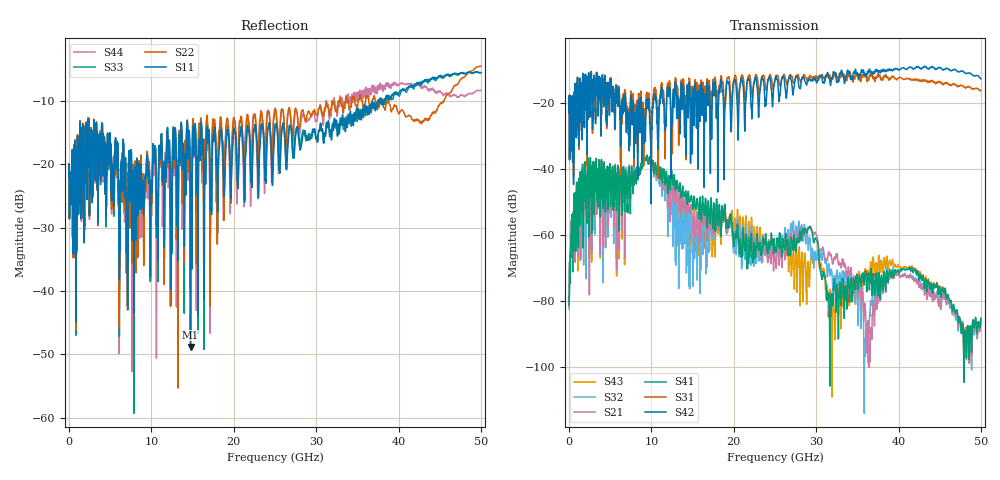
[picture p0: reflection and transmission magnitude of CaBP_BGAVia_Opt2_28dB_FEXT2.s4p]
!* Samtec Inc. NovaRay Examax Flyover System  *
!*  REV DATE  = 08/08/18  *
!*  TYPE  = TOUCHSTONE  *
!*  PORTS  = 4 port  *
!*  UNITS  = GHz  *
!*  DATA RANGE = DC  to 50 GHz; 10 MHz Step  *
!*  PARAMETER  = S  *
!*  FORMAT  = Real-Imaginary  *
!*  REFERENCE  = 50 ohms  *
!*  SOURCE  = HFSS  *
!*  VALIDATED  = No  *
!*  MANUFACTURER = SAMTEC  *
!*  INTERCONNECT = NVAx to EBCx to EBCx to NVAx  *
!*  [Full Channel NVAx to EBCx to EBCx to NVAx  with PCB Trace and BGA Via]  *
!*  BOUNDARY A  = Silicon BGA Ball Pad  *
!*  BOUNDARY B  = Silicon BGA Ball Pad  *
!*  NVAx (end a) ->>- (end b) NVAx  *
!*  Port 01 ->>- Port 02  *
!*  Port 03 ->>- Port 04  *
!***************************** CHANNEL MODEL ******************************************
# GHz S RI R 50
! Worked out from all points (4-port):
!   5000 points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, 10 MHz to 50 GHz, reference 50 ohm
!   strongest paths, dB at 10 MHz, 12.51 GHz, 25.01 GHz, 37.51 GHz, 50 GHz:
!     S42: -23.1, -26.3, -12.7, -10.5, -12.7
!     S31: -23.1, -28.5, -13.0, -11.3, -16.4
!     S41: -81.3, -42.6, -64.0, -77.3, -85.4
!     S21: -82.1, -46.0, -67.1, -78.8, -86.3
!     S32: -82.7, -51.9, -65.2, -75.4, -86.3
!     S43: -81.6, -46.4, -64.4, -70.1, -85.3
!   lowest |S11| = -48.8 dB at 14.75 GHz (marker M1), VSWR 1.01, Z = 49.7 - j0.221 ohm
!   |S11| at or under -10 dB: start of sweep to 37.51 GHz; 37.83997 GHz to 38.00552 GHz (165.6 MHz wide, 0.437 % of centre); 38.04261 GHz to 38.22467 GHz (182.1 MHz wide, 0.477 % of centre)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
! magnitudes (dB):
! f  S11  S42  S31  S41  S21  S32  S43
! 10 MHz  -22.1  -23.1  -23.1  -81.3  -82.1  -82.7  -81.6
! 1.43 GHz  -14.9  -13.9  -13.8  -48.1  -50.2  -52.2  -50.2
! 9.26 GHz  -21.6  -31.8  -26.8  -37.1  -37.3  -37.3  -37.0
! 14.75 GHz  -48.8  -38.3  -22.0  -49.3  -51.7  -56.3  -55.7
! 29.25 GHz  -16.1  -12.7  -11.7  -57.6  -57.7  -61.1  -71.4
! 31.79 GHz  -15.2  -14.1  -13.4  -78.6  -66.1  -71.1  -78.7
! 50 GHz  -5.6  -12.7  -16.4  -85.4  -86.3  -86.3  -85.3
